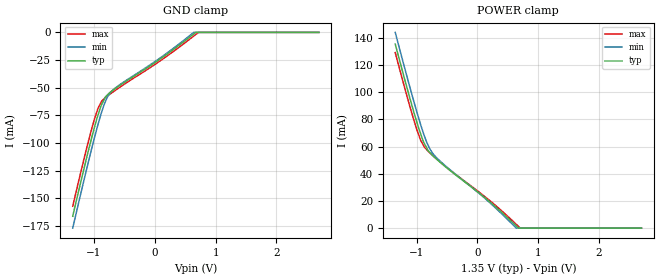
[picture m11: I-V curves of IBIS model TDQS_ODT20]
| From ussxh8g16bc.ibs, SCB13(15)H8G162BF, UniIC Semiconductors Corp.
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| MODEL TDQS_ODT20 (TDQS Terminator Model with 20ohm ODT, 800-2133Mbps)
[Model]   TDQS_ODT20
Model_type   Terminator
|   typ   min   max
|C_comp   1.035pF   0.986pF   1.103pF
C_comp_power_clamp   0.5175pF   0.4930pF   0.5515pF
C_comp_gnd_clamp   0.5175pF   0.4930pF   0.5515pF
| Note: C_comp changes when the ODT circuit is enabled.
[Voltage Range]   1.3500V   1.2830V   1.4250V
| Junction Temperature (Ambient temp is 40C typ, 85C min, 0C max)
[Temperature Range]   45.0   90.0   0.0
[GND Clamp]
|   Voltage   I(typ)   I(min)   I(max)
-1.35V    -166.3mA   -177.1mA   -157.3mA
-1.11V    -110.8mA   -121mA     -102.3mA
-990mV    -85.35mA   -94.61mA   -77.81mA
-935mV    -74.97mA   -83.31mA   -68.79mA
-885mV    -66.4mA    -73.78mA   -63.4mA
-810mV    -58.2mA    -62.2mA    -58.78mA
-785mV    -56.84mA   -58.97mA   -57.76mA
-680mV    -51.97mA   -51.62mA   -53.61mA
110mV     -23.21mA   -22.26mA   -24.93mA
640mV     -1.463mA   0A         -3.331mA
718mV     0A         0A         0A
2.7V      0A         0A         0A
[POWER Clamp]
|   Voltage   I(typ)   I(min)   I(max)
-1.35V    135.5mA    144.1mA    129.2mA
-1.11V    95.68mA    103.8mA    89.59mA
-990mV    77.3mA     84.75mA    71.78mA
-930mV    69.11mA    75.86mA    64.5mA
-885mV    63.46mA    69.61mA    60.78mA
-780mV    55.58mA    58.21mA    55.37mA
-730mV    53.18mA    54.8mA     53.36mA
-590mV    47.64mA    48.4mA     47.94mA
115mV     22.74mA    22.32mA    23.5mA
640mV     1.535mA    94.48uA    2.842mA
707mV     0A         0A         0A
2.7V      0A         0A         0A
